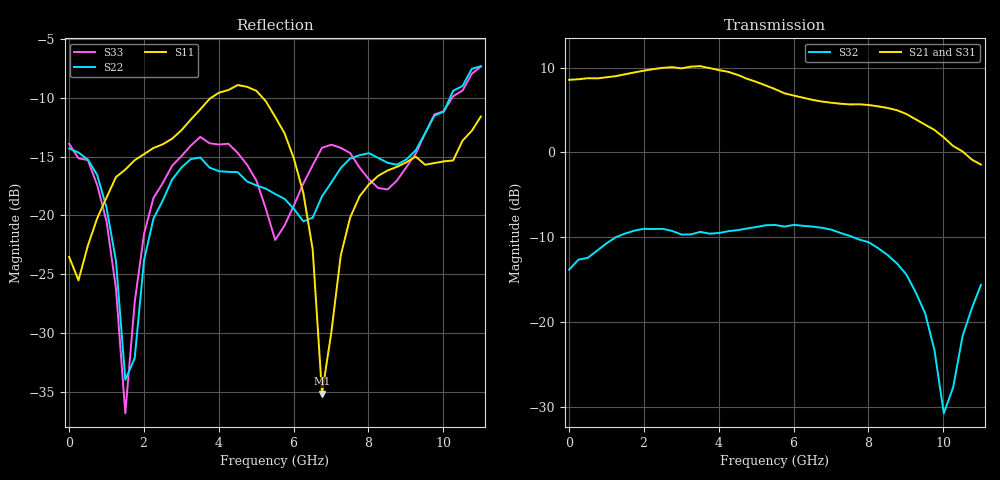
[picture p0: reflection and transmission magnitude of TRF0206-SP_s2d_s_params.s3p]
! Created Wed Sep 28 01:20:20 2022
# hz S ri R 50
! 3 Port Network Data from SP1.SP block
! freq  reS11  imS11  reS12  imS12  reS13  imS13
!  reS21  imS21
!  reS22  imS22  reS23  imS23
!  reS31  imS31  reS32  imS32
!  reS33  imS33
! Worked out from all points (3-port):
!   45 points, 10 MHz to 11 GHz, reference 50 ohm
!   strongest paths, dB at 10 MHz, 2.76 GHz, 5.51 GHz, 8.26 GHz, 11 GHz:
!     S21: 8.6, 10.0, 7.5, 5.4, -1.4
!     S31: 8.5, 10.0, 7.3, 5.2, -1.8
!     S32: -13.8, -9.3, -8.6, -11.3, -15.6
!   lowest |S11| = -35.2 dB at 6.76 GHz (marker M1), VSWR 1.04, Z = 49.4 - j1.62 ohm
!   |S11| at or under -10 dB: start of sweep to 3.793 GHz; 5.182 GHz to end of sweep
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1e7  0.0588 -0.0312  -0.0549 0.00231  -0.0419 0.000467
     2.677 0.0721  -0.1922 -0.0132  0.2216 0.0136
     -2.646 0.0192  0.2036 0.00473  -0.2008 0.0203
1.51e9  -0.0466 -0.1497  -0.06 0.0366  -0.0491 0.0371
        1.659 -2.363  -0.0139 0.0143  0.2694 -0.1706
        -1.664 2.374  0.2875 -0.1675  0.012 0.00785
2.51e9  -0.0897 -0.1797  -0.0301 0.0655  -0.0141 0.0584
        -0.3348 -3.134  -0.00957 -0.1154  0.0604 -0.3166
        0.3875 3.133  0.0711 -0.3473  -0.0114 -0.1369
3.26e9  -0.0678 -0.247  -0.00582 0.0689  0.0111 0.0534
        -2.007 -2.494  -0.0508 -0.1662  -0.1253 -0.2661
        2.043 2.408  -0.1363 -0.299  -0.0688 -0.1862
4.01e9  -0.0752 -0.3246  0.0207 0.0673  0.0296 0.041
        -2.943 -0.8214  -0.0624 -0.1411  -0.2621 -0.1386
        2.893 0.776  -0.2983 -0.1523  -0.1238 -0.1575
5.51e9  -0.1008 -0.2427  0.063 0.0373  0.0468 0.0119
        -1.631 1.703  -0.0201 -0.1217  -0.3058 0.1548
        1.596 -1.68  -0.3067 0.2131  -0.0157 -0.0771
6.76e9  -0.00594 -0.0164  0.0709 -0.0129  0.0393 -0.0266
        -0.0256 1.993  0.1142 -0.0388  -0.1606 0.3544
        0.00787 -1.945  -0.1036 0.3442  0.1892 -0.0433
8.76e9  0.145 0.0699  0.0117 -0.0606  -0.0125 -0.0202
        1.772 -0.000772  0.0885 -0.1385  0.1846 0.1231
        -1.721 0.0545  0.149 0.1641  0.034 -0.1366
1.001e10  0.1388 -0.098  -0.0313 -0.034  -0.0081 -0.00109
          0.4929 -1.122  -0.0783 -0.2653  -0.00696 -0.0178
          -0.477 1.111  0.0209 -0.0202  -0.0139 -0.2776
1.1e10  0.00971 -0.2636  -0.0306 -0.0136  -0.00136 -0.00188
        -0.258 -0.8078  -0.2208 -0.3712  -0.1612 0.0678
        0.3193 0.7469  -0.1566 0.053  -0.2949 -0.313
